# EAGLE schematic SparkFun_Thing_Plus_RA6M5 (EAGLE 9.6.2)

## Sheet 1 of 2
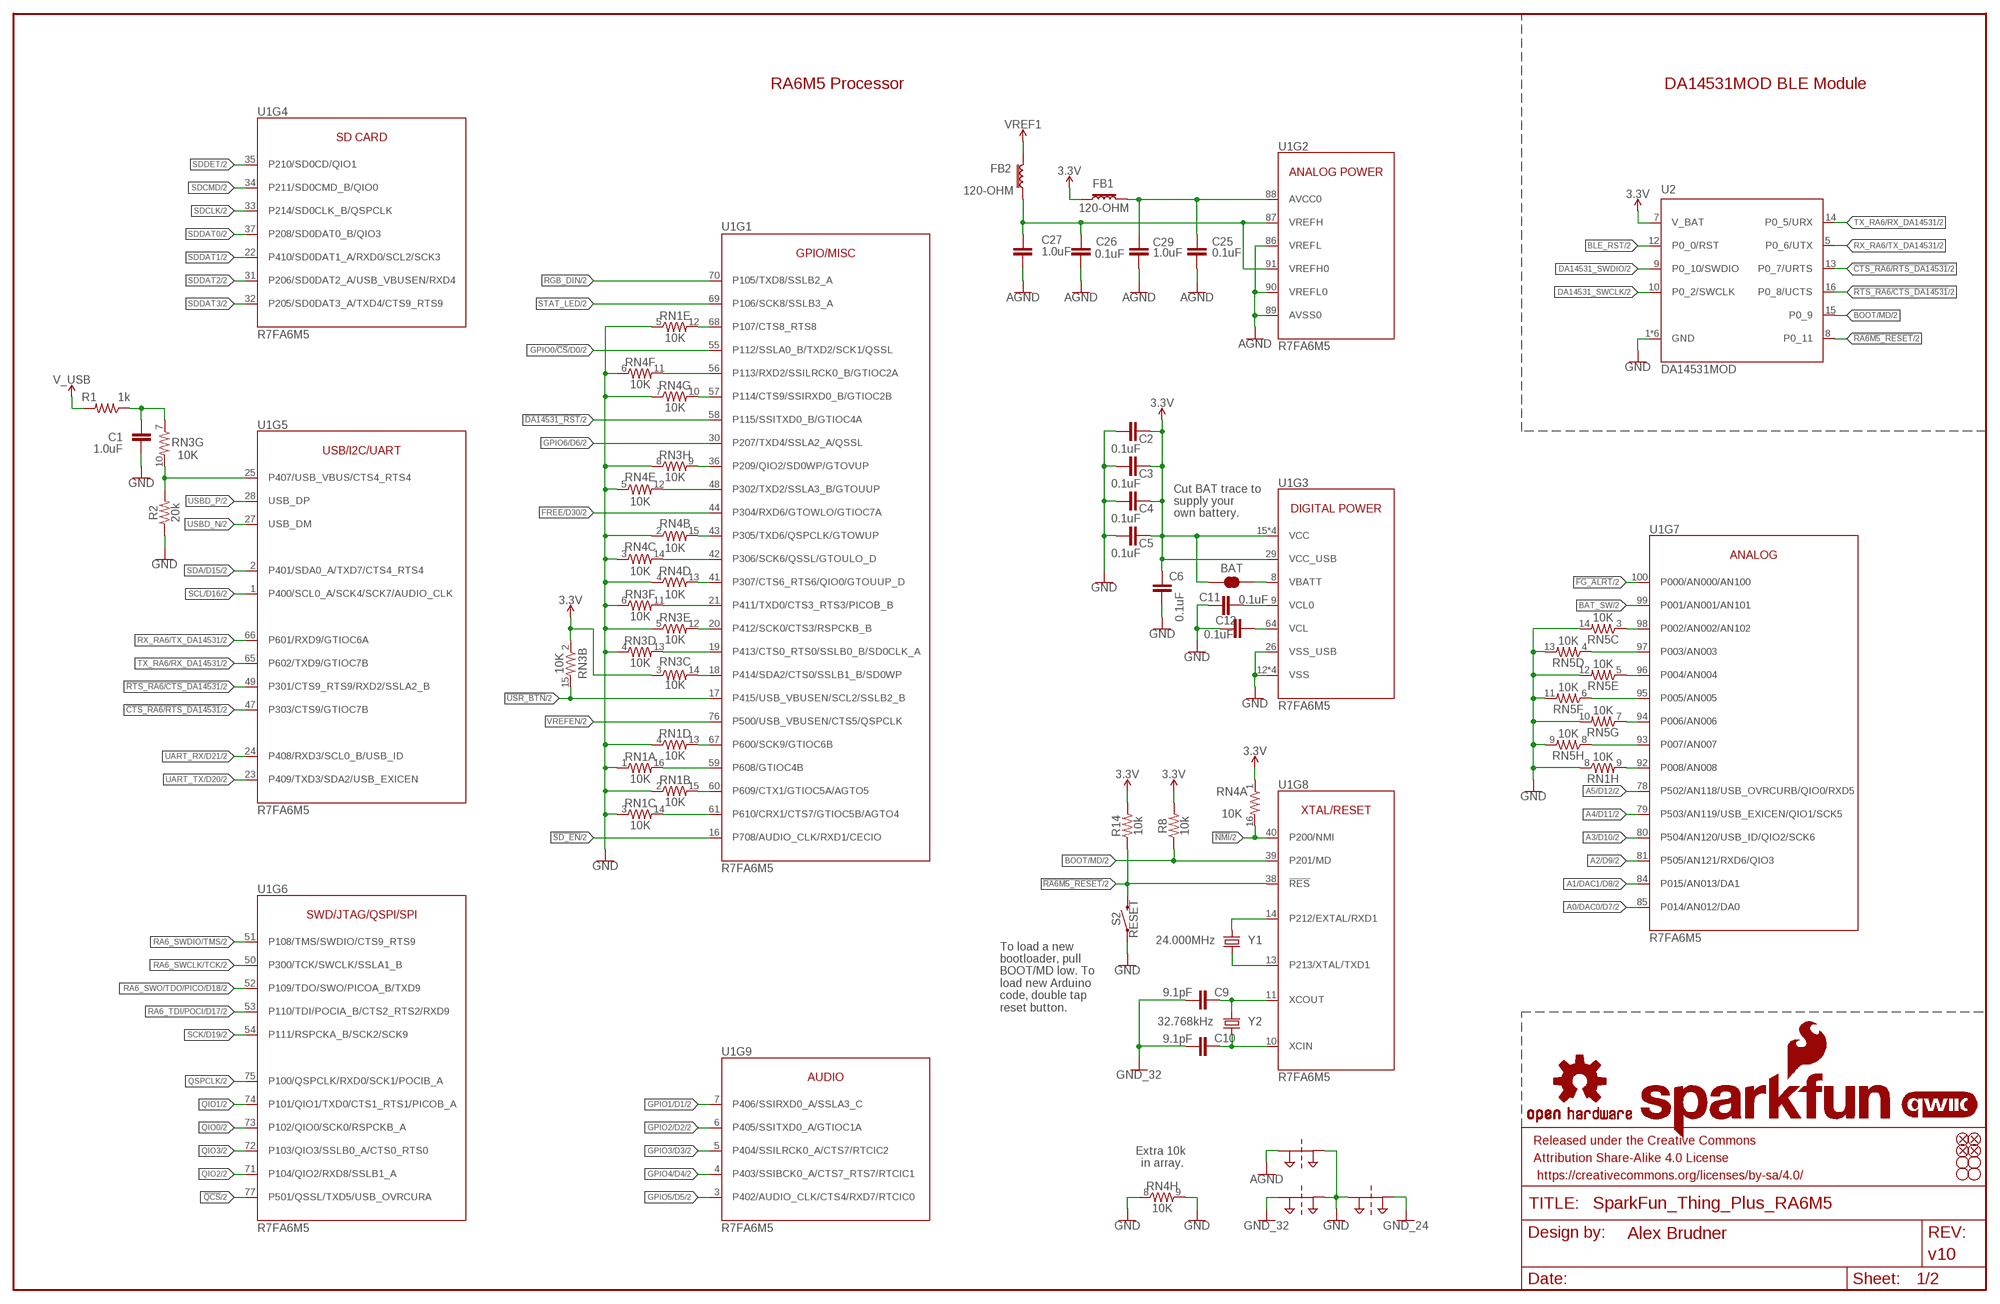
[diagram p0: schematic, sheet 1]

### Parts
BAT  JUMPER-SMT_2_NC_TRACE_SILK  [SMT-JUMPER_2_NC_TRACE_SILK]
C1  1.0uF  1.0UF-0402T-16V-10%  [0402-TIGHT]
C2  0.1uF  0.1UF-0402T-16V-10%  [0402-TIGHT]
C3  0.1uF  0.1UF-0402T-16V-10%  [0402-TIGHT]
C4  0.1uF  0.1UF-0402T-16V-10%  [0402-TIGHT]
C5  0.1uF  0.1UF-0402T-16V-10%  [0402-TIGHT]
C6  0.1uF  0.1UF-0402T-16V-10%  [0402-TIGHT]
C9  9.1pF  9.1PF-0402-TIGHT  [0402-TIGHT]
C10  9.1pF  9.1PF-0402-TIGHT  [0402-TIGHT]
C11  0.1uF  0.1UF-0402T-16V-10%  [0402-TIGHT]
C12  0.1uF  0.1UF-0402T-16V-10%  [0402-TIGHT]
C25  0.1uF  0.1UF-0402T-16V-10%  [0402-TIGHT]
C26  0.1uF  0.1UF-0402T-16V-10%  [0402-TIGHT]
C27  1.0uF  1.0UF-0402T-16V-10%  [0402-TIGHT]
C29  1.0uF  1.0UF-0402T-16V-10%  [0402-TIGHT]
FB1  120-OHM  FERRITE_BEAD-120_OHM-0402T  [0402-TIGHT]
FB2  120-OHM  FERRITE_BEAD-120_OHM-0402T  [0402-TIGHT]
FD1  FIDUCIALUFIDUCIAL  [FIDUCIAL-MICRO]
FD2  FIDUCIALUFIDUCIAL  [FIDUCIAL-MICRO]
FD3  FIDUCIALUFIDUCIAL  [FIDUCIAL-MICRO]
FD4  FIDUCIALUFIDUCIAL  [FIDUCIAL-MICRO]
FRAME1  FRAME-LEDGER  [CREATIVE_COMMONS]
H1  STAND-OFFTIGHT  [STAND-OFF-TIGHT]
H2  STAND-OFFTIGHT  [STAND-OFF-TIGHT]
H3  STAND-OFFTIGHT  [STAND-OFF-TIGHT]
H4  STAND-OFFTIGHT  [STAND-OFF-TIGHT]
LOGO1  OSHW-LOGOMINI  [OSHW-LOGO-MINI]
LOGO2  SFE_LOGO_NAME_FLAME.1_INCH  [SFE_LOGO_NAME_FLAME_.1]
LOGO3  QWIIC_LOGO_4MM  [QWIIC_4MM]
R1  1k  1KOHM-0402T-1/16W-1%  [0402-TIGHT]
R2  20k  20KOHM-0402T-1/16W-1%  [0402-TIGHT]
R8  10k  10KOHM-0402T-1/16W-1%  [0402-TIGHT]
R14  10k  10KOHM-0402T-1/16W-1%  [0402-TIGHT]
RN1  10K  10KOHM-ARRAY(8)-2506_ARV-1/16W-5%  [2506_AR]
RN3  10K  10KOHM-ARRAY(8)-2506_ARV-1/16W-5%  [2506_AR]
RN4  10K  10KOHM-ARRAY(8)-2506_ARV-1/16W-5%  [2506_AR]
RN5  10K  10KOHM-ARRAY(8)-2506_ARV-1/16W-5%  [2506_AR]
S2  RESET  MOMENTARY-SWITCH-SPST-SMD-4.6X2.8MM  [TACTILE_SWITCH_SMD_4.6X2.8MM]
SUPPLYTIE1  2PT_GND_TIESMALL  [2PT_GND_TIE_SMALL]
SUPPLYTIE2  2PT_GND_TIESMALL  [2PT_GND_TIE_SMALL]
SUPPLYTIE3  2PT_GND_TIESMALL  [2PT_GND_TIE_SMALL]
U1  R7FA6M5  R7FA6M5-100LQFP  [P-LQFP100-14X14-0.50]
U2  DA14531MOD  [DA14531MOD]
Y1  24.000MHz  CRYSTAL-24.000MHZ-8PF-4-SMD  [4-SMD,32X25]
Y2  32.768kHz  CRYSTAL-32.768KHZSMD-3.2X1.5  [CRYSTAL-SMD-3.2X1.5MM]

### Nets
3.3V [Power]: BAT.1 C2.1 C3.1 C4.1 C5.1 C6.1 FB1.1 R8.2 R14.2 RN3.2 RN3.3 RN4.1 U1.15(VCC) U1.29(VCC_USB) U1.46(VCC) U1.62(VCC) U1.82(VCC) U2.7(V_BAT) ; also sheet 2
!CTS_RA6/RTS_DA14531! [LS Digital]: U1.47(P303/CTS9/GTIOC7B) U2.13(P0_7/URTS) ; also sheet 2
!DA14531_RST!: U1.58(P115/SSITXD0_B/GTIOC4A) ; also sheet 2
!FG_ALRT!: U1.100(P000/AN000/AN100) ; also sheet 2
!NMI!: RN4.16 U1.40(P200/NMI) ; also sheet 2
!QCS!: U1.77(P501/QSSL/TXD5/USB_OVRCURA) ; also sheet 2
!RA6M5_RESET!: R14.1 S2.3 S2.4 U1.38(!RES!) U2.8(P0_11) ; also sheet 2
!RTS_RA6/CTS_DA14531! [LS Digital]: U1.49(P301/CTS9_RTS9/RXD2/SSLA2_B) U2.16(P0_8/UCTS) ; also sheet 2
!SD_EN!: U1.16(P708/AUDIO_CLK/RXD1/CECIO) ; also sheet 2
!USR_BTN!: RN3.15 U1.17(P415/USB_VBUSEN/SCL2/SSLB2_B) ; also sheet 2
A0/DAC0/D7 [Analog]: U1.85(P014/AN012/DA0) ; also sheet 2
A1/DAC1/D8 [Analog]: U1.84(P015/AN013/DA1) ; also sheet 2
A2/D9 [Analog]: U1.81(P505/AN121/RXD6/QIO3) ; also sheet 2
A3/D10 [Analog]: U1.80(P504/AN120/USB_ID/QIO2/SCK6) ; also sheet 2
A4/D11 [Analog]: U1.79(P503/AN119/USB_EXICEN/QIO1/SCK5) ; also sheet 2
A5/D12 [Analog]: U1.78(P502/AN118/USB_OVRCURB/QIO0/RXD5) ; also sheet 2
AGND [Analog Ground]: C25.2 C26.2 C27.2 C29.2 SUPPLYTIE1.P$1 U1.86(VREFL) U1.89(AVSS0) U1.90(VREFL0)
AVCC0 [Power]: C25.1 C29.1 FB1.2 U1.88(AVCC0) ; also sheet 2
BAT_SW: U1.99(P001/AN001/AN101) ; also sheet 2
BLE_RST: U2.12(P0_0/RST) ; also sheet 2
BOOT/MD: R8.1 U1.39(P201/MD) U2.15(P0_9) ; also sheet 2
DA14531_SWCLK [HS Digital]: U2.10(P0_2/SWCLK) ; also sheet 2
DA14531_SWDIO [HS Digital]: U2.9(P0_10/SWDIO) ; also sheet 2
EXTAL [CLK signals]: U1.14(P212/EXTAL/RXD1) Y1.1
FREE/D30: U1.44(P304/RXD6/GTOWLO/GTIOC7A) ; also sheet 2
GND [Power]: C1.1 C2.2 C3.2 C4.2 C5.2 C6.2 C11.2 C12.2 R2.1 RN1.1 RN1.2 RN1.3 RN1.4 RN1.5 RN1.8 RN3.4 RN3.5 RN3.6 RN3.8 RN4.2 RN4.3 RN4.4 RN4.5 RN4.6 RN4.7 RN4.8 RN4.9 RN5.9 RN5.10 RN5.11 RN5.12 RN5.13 RN5.14 S2.1 S2.2 SUPPLYTIE1.P$2 SUPPLYTIE2.P$2 SUPPLYTIE3.P$1 U1.12(VSS) U1.26(VSS_USB) U1.45(VSS) U1.63(VSS) U1.83(VSS) U2.1(GND) U2.2(GND) U2.3(GND) U2.4(GND) U2.6(GND) U2.11(GND) ; also sheet 2
GND_24 [CLK grounds]: SUPPLYTIE3.P$2
GND_32 [CLK grounds]: C9.1 C10.1 SUPPLYTIE2.P$1
GPIO0/!CS!/D0: U1.55(P112/SSLA0_B/TXD2/SCK1/QSSL) ; also sheet 2
GPIO1/D1: U1.7(P406/SSIRXD0_A/SSLA3_C) ; also sheet 2
GPIO2/D2: U1.6(P405/SSITXD0_A/GTIOC1A) ; also sheet 2
GPIO3/D3: U1.5(P404/SSILRCK0_A/CTS7/RTCIC2) ; also sheet 2
GPIO4/D4: U1.4(P403/SSIBCK0_A/CTS7_RTS7/RTCIC1) ; also sheet 2
GPIO5/D5: U1.3(P402/AUDIO_CLK/CTS4/RXD7/RTCIC0) ; also sheet 2
GPIO6/D6: U1.30(P207/TXD4/SSLA2_A/QSSL) ; also sheet 2
N$7: RN1.9 U1.92(P008/AN008)
N$8: RN3.9 U1.36(P209/QIO2/SD0WP/GTOVUP)
N$9: C1.2 R1.1 RN3.7
N$13: RN3.14 U1.18(P414/SDA2/CTS0/SSLB1_B/SD0WP)
N$15: R2.2 RN3.10 U1.25(P407/USB_VBUS/CTS4_RTS4)
N$17: RN1.14 U1.61(P610/CRX1/CTS7/GTIOC5B/AGTO4)
N$18: RN1.15 U1.60(P609/CTX1/GTIOC5A/AGTO5)
N$22: RN1.16 U1.59(P608/GTIOC4B)
N$23: RN4.15 U1.43(P305/TXD6/QSPCLK/GTOWUP)
N$24: RN1.13 U1.67(P600/SCK9/GTIOC6B)
N$26: RN3.13 U1.19(P413/CTS0_RTS0/SSLB0_B/SD0CLK_A)
N$27: RN3.12 U1.20(P412/SCK0/CTS3/RSPCKB_B)
N$28: RN3.11 U1.21(P411/TXD0/CTS3_RTS3/PICOB_B)
N$29 [Power]: C26.1 C27.1 FB2.1 U1.87(VREFH) U1.91(VREFH0)
N$30: RN4.13 U1.41(P307/CTS6_RTS6/QIO0/GTOUUP_D)
N$31: RN4.12 U1.48(P302/TXD2/SSLA3_B/GTOUUP)
N$32: RN4.14 U1.42(P306/SCK6/QSSL/GTOULO_D)
N$33 [Power]: BAT.2 U1.8(VBATT)
N$35: RN4.10 U1.57(P114/CTS9/SSIRXD0_B/GTIOC2B)
N$36: RN4.11 U1.56(P113/RXD2/SSILRCK0_B/GTIOC2A)
N$37: RN1.12 U1.68(P107/CTS8_RTS8)
N$41: RN5.8 U1.93(P007/AN007)
N$42: RN5.7 U1.94(P006/AN006)
N$43: RN5.6 U1.95(P005/AN005)
N$44: RN5.5 U1.96(P004/AN004)
N$45: RN5.4 U1.97(P003/AN003)
N$46: RN5.3 U1.98(P002/AN002/AN102)
N$97: C11.1 U1.9(VCL0)
N$98: C12.1 U1.64(VCL)
QIO0 [HS Digital]: U1.73(P102/QIO0/SCK0/RSPCKB_A) ; also sheet 2
QIO1 [HS Digital]: U1.74(P101/QIO1/TXD0/CTS1_RTS1/PICOB_A) ; also sheet 2
QIO2 [HS Digital]: U1.71(P104/QIO2/RXD8/SSLB1_A) ; also sheet 2
QIO3 [HS Digital]: U1.72(P103/QIO3/SSLB0_A/CTS0_RTS0) ; also sheet 2
QSPCLK [HS Digital]: U1.75(P100/QSPCLK/RXD0/SCK1/POCIB_A) ; also sheet 2
RA6_SWCLK/TCK [HS Digital]: U1.50(P300/TCK/SWCLK/SSLA1_B) ; also sheet 2
RA6_SWDIO/TMS [HS Digital]: U1.51(P108/TMS/SWDIO/CTS9_RTS9) ; also sheet 2
RA6_SWO/TDO/PICO/D18 [HS Digital]: U1.52(P109/TDO/SWO/PICOA_B/TXD9) ; also sheet 2
RA6_TDI/POCI/D17 [HS Digital]: U1.53(P110/TDI/POCIA_B/CTS2_RTS2/RXD9) ; also sheet 2
RGB_DIN [LS Digital]: U1.70(P105/TXD8/SSLB2_A) ; also sheet 2
RX_RA6/TX_DA14531 [LS Digital]: U1.66(P601/RXD9/GTIOC6A) U2.5(P0_6/UTX) ; also sheet 2
SCK/D19 [HS Digital]: U1.54(P111/RSPCKA_B/SCK2/SCK9) ; also sheet 2
SCL/D16 [LS Digital]: U1.1(P400/SCL0_A/SCK4/SCK7/AUDIO_CLK) ; also sheet 2
SDA/D15 [LS Digital]: U1.2(P401/SDA0_A/TXD7/CTS4_RTS4) ; also sheet 2
SDCLK [HS Digital]: U1.33(P214/SD0CLK_B/QSPCLK) ; also sheet 2
SDCMD [LS Digital]: U1.34(P211/SD0CMD_B/QIO0) ; also sheet 2
SDDAT0 [HS Digital]: U1.37(P208/SD0DAT0_B/QIO3) ; also sheet 2
SDDAT1 [HS Digital]: U1.22(P410/SD0DAT1_A/RXD0/SCL2/SCK3) ; also sheet 2
SDDAT2 [HS Digital]: U1.31(P206/SD0DAT2_A/USB_VBUSEN/RXD4) ; also sheet 2
SDDAT3 [HS Digital]: U1.32(P205/SD0DAT3_A/TXD4/CTS9_RTS9) ; also sheet 2
SDDET: U1.35(P210/SD0CD/QIO1) ; also sheet 2
STAT_LED: U1.69(P106/SCK8/SSLB3_A) ; also sheet 2
TX_RA6/RX_DA14531 [LS Digital]: U1.65(P602/TXD9/GTIOC7B) U2.14(P0_5/URX) ; also sheet 2
UART_RX/D21 [LS Digital]: U1.24(P408/RXD3/SCL0_B/USB_ID) ; also sheet 2
UART_TX/D20 [LS Digital]: U1.23(P409/TXD3/SDA2/USB_EXICEN) ; also sheet 2
USBD_N [USB diff]: U1.27(USB_DM) ; also sheet 2
USBD_P [USB diff]: U1.28(USB_DP) ; also sheet 2
V_USB [Power]: R1.2 ; also sheet 2
VREF1 [Power]: FB2.2 ; also sheet 2
VREFEN: U1.76(P500/USB_VBUSEN/CTS5/QSPCLK) ; also sheet 2
XCIN [CLK signals]: C10.2 U1.10(XCIN) Y2.P$1
XCOUT [CLK signals]: C9.2 U1.11(XCOUT) Y2.P$2
XTAL [CLK signals]: U1.13(P213/XTAL/TXD1) Y1.3

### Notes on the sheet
- RA6M5 Processor | DA14531MOD BLE Module
- Cut BAT trace to 
  supply your 
  own battery.
- To load a new 
  bootloader, pull 
  BOOT/MD low. To 
  load new Arduino 
  code, double tap 
  reset button.
- Extra 10k 
  in array.

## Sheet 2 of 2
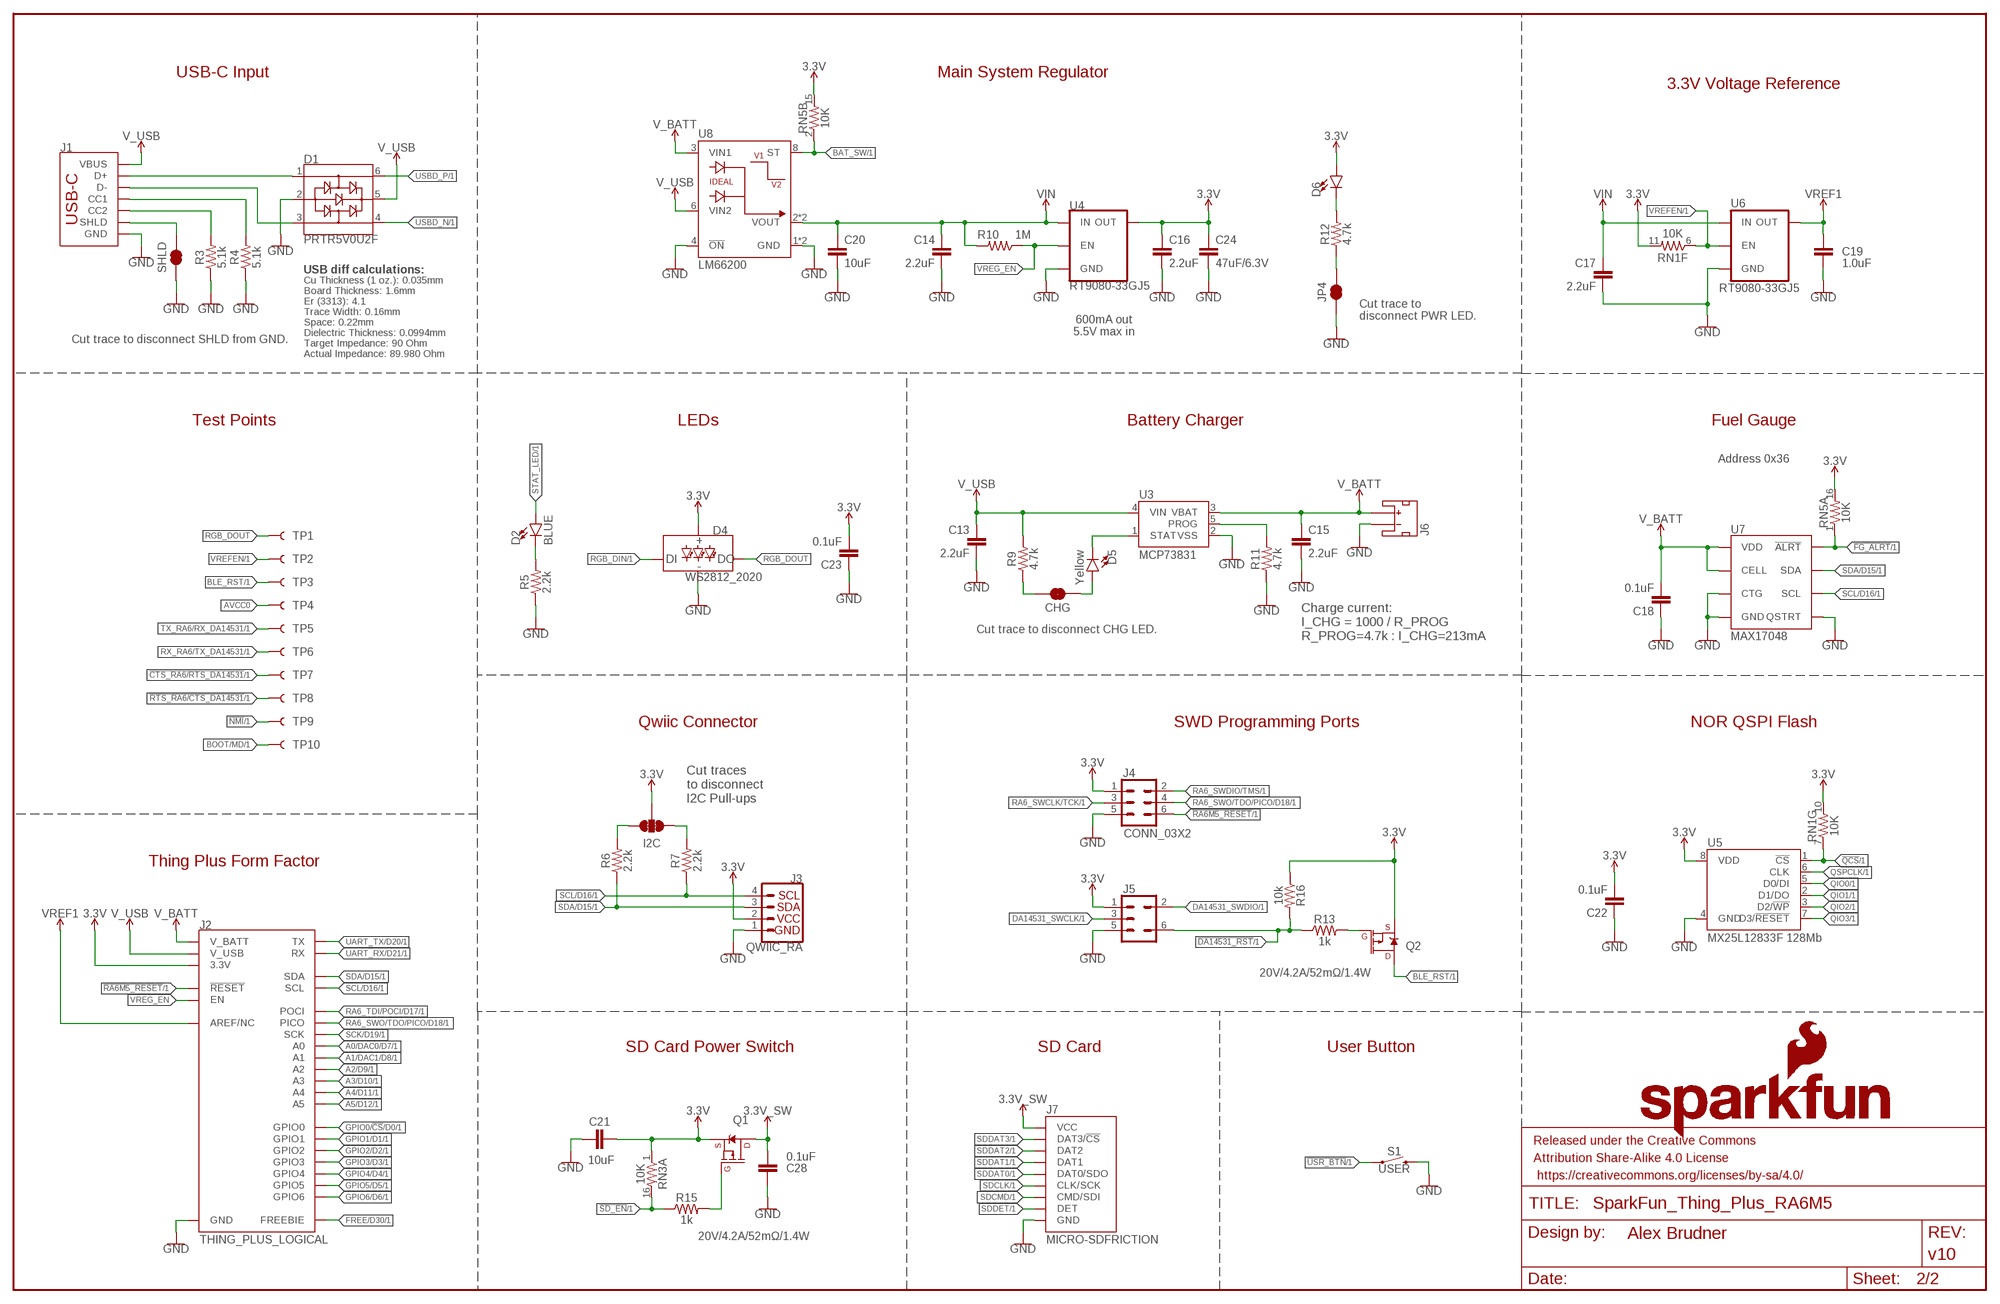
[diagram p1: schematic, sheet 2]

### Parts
C13  2.2uF  2.2UF-0402_TIGHT-10V-10%-X5R  [0402-TIGHT]
C14  2.2uF  2.2UF-0402_TIGHT-10V-10%-X5R  [0402-TIGHT]
C15  2.2uF  2.2UF-0402_TIGHT-10V-10%-X5R  [0402-TIGHT]
C16  2.2uF  2.2UF-0402_TIGHT-10V-10%-X5R  [0402-TIGHT]
C17  2.2uF  2.2UF-0402_TIGHT-10V-10%-X5R  [0402-TIGHT]
C18  0.1uF  0.1UF-0402T-16V-10%  [0402-TIGHT]
C19  1.0uF  1.0UF-0402T-16V-10%  [0402-TIGHT]
C20  10uF  10UF-0805-25V-10%  [0805]
C21  10uF  10UF-0805-25V-10%  [0805]
C22  0.1uF  0.1UF-0402T-16V-10%  [0402-TIGHT]
C23  0.1uF  0.1UF-0402T-16V-10%  [0402-TIGHT]
C24  47uF/6.3V  47UF  [0805]
C28  0.1uF  0.1UF-0402T-16V-10%  [0402-TIGHT]
CHG  JUMPER-SMT_2_NC_TRACE_SILK  [SMT-JUMPER_2_NC_TRACE_SILK]
D1  PRTR5V0U2F  [SOT886]
D2  BLUE  LED-BLUE0603  [LED-0603]
D4  WS2812_2020  [WS2812-2020]
D5  Yellow  LED-YELLOW0603  [LED-0603]
D6  LED-RED_0603-KB  [LED-0603]
FRAME2  FRAME-LEDGERNO_FOOTPRINT  [DUMMY]
I2C  JUMPER-SMT_3_2-NC_TRACE_SILK  [SMT-JUMPER_3_2-NC_TRACE_SILK]
J1  USB Female Type C Connector  USB_C_6-LAYER-ISOLATED  [USB-C-16P-6LAYER-ISOLATED]
J2  THING_PLUS_LOGICAL  [THING_PLUS]
J3  QWIIC_RA  QWIIC_CONNECTORJS-1MM  [JST04_1MM_RA]
J4  CONN_03X2  [PAD_05_03X2_TP]
J5  SWD-5PIN  [PAD_05_03X2_TP_NO4]
J6  JST_2MM_MALE  [JST-2-SMD]
J7  MICRO-SDFRICTION  [MICROSD_TINY]
JP4  JUMPER-SMT_2_NC_TRACE_SILK  [SMT-JUMPER_2_NC_TRACE_SILK]
LOGO4  SFE_LOGO_NAME_FLAMEBLANK  [BLANK]
Q1  20V/4.2A/52mΩ/1.4W  MOSFET_PCH-DMG2305UX-7  [SOT23-3]
Q2  20V/4.2A/52mΩ/1.4W  MOSFET_PCH-DMG2305UX-7  [SOT23-3]
R3  5.1k  5.1KOHM-0402T-1/16W-1%  [0402-TIGHT]
R4  5.1k  5.1KOHM-0402T-1/16W-1%  [0402-TIGHT]
R5  2.2k  2.2KOHM-0402T-1/16W-1%  [0402-TIGHT]
R6  2.2k  2.2KOHM-0402T-1/16W-1%  [0402-TIGHT]
R7  2.2k  2.2KOHM-0402T-1/16W-1%  [0402-TIGHT]
R9  4.7k  4.7KOHM-0402T-1/16W-1%  [0402-TIGHT]
R10  1M  1MOHM-0402T-1/16W-5%  [0402-TIGHT]
R11  4.7k  4.7KOHM-0402T-1/16W-1%  [0402-TIGHT]
R12  4.7k  4.7KOHM-0402T-1/16W-1%  [0402-TIGHT]
R13  1k  1KOHM-0402T-1/16W-1%  [0402-TIGHT]
R15  1k  1KOHM-0402T-1/16W-1%  [0402-TIGHT]
R16  10k  10KOHM-0402T-1/16W-1%  [0402-TIGHT]
S1  USER  MOMENTARY-SWITCH-SPST-SMD-4.6X2.8MM  [TACTILE_SWITCH_SMD_4.6X2.8MM]
SHLD  JUMPER-SMT_2_NC_TRACE_SILK  [SMT-JUMPER_2_NC_TRACE_SILK]
TP1  TEST-POINT3X5  [PAD.03X.05]
TP2  TEST-POINT3X4  [PAD.03X.04]
TP3  TEST-POINT3X5  [PAD.03X.05]
TP4  TEST-POINT3  [PAD.03X.03]
TP5  TEST-POINT3X5  [PAD.03X.05]
TP6  TEST-POINT3X5  [PAD.03X.05]
TP7  TEST-POINT3X5  [PAD.03X.05]
TP8  TEST-POINT3X5  [PAD.03X.05]
TP9  TEST-POINT3  [PAD.03X.03]
TP10  TEST-POINT3X5  [PAD.03X.05]
U3  MCP73831  [SOT23-5]
U4  RT9080-33GJ5  V_REG_RT9080  [SOT23-5]
U5  MX25L12833F 128Mb  MX25L12833F_128MBIT_QSPI  [WSON-8-6X5]
U6  RT9080-33GJ5  V_REG_RT9080  [SOT23-5]
U7  MAX17048  MAX17048DFN8  [DFN-8]
U8  LM66200  IDEAL_DIODE_DUAL_LM66200  [SOT8]

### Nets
3.3V [Power]: C16.1 C21.1 C22.2 C23.2 C24.1 D4.VCC D6.A I2C.2 J2.27(3.3V) J3.2 J4.1 J5.1 Q1.2(S) Q2.2(S) R16.1 RN1.10 RN1.11 RN3.1 RN5.15 RN5.16 U4.5(OUT) U5.8(VDD) ; also sheet 1
3.3V_SW [Power]: C28.2 J7.4(VCC) Q1.3(D)
!CTS_RA6/RTS_DA14531! [LS Digital]: TP7.1 ; also sheet 1
!DA14531_RST!: J5.6 R13.1 R16.2 ; also sheet 1
!FG_ALRT!: RN5.1 U7.5(!ALRT) ; also sheet 1
!NMI!: TP9.1 ; also sheet 1
!QCS!: RN1.7 U5.1(!CS!) ; also sheet 1
!RA6M5_RESET!: J2.28(!RESET) J4.6 ; also sheet 1
!RTS_RA6/CTS_DA14531! [LS Digital]: TP8.1 ; also sheet 1
!SD_EN!: R15.1 RN3.16 ; also sheet 1
!USR_BTN!: S1.1 S1.2 ; also sheet 1
A0/DAC0/D7 [Analog]: J2.24(A0) ; also sheet 1
A1/DAC1/D8 [Analog]: J2.23(A1) ; also sheet 1
A2/D9 [Analog]: J2.22(A2) ; also sheet 1
A3/D10 [Analog]: J2.21(A3) ; also sheet 1
A4/D11 [Analog]: J2.20(A4) ; also sheet 1
A5/D12 [Analog]: J2.19(A5) ; also sheet 1
AVCC0 [Power]: TP4.1 ; also sheet 1
BAT_SW: RN5.2 U8.8(ST) ; also sheet 1
BLE_RST: Q2.3(D) TP3.1 ; also sheet 1
BOOT/MD: TP10.1 ; also sheet 1
DA14531_SWCLK [HS Digital]: J5.3 ; also sheet 1
DA14531_SWDIO [HS Digital]: J5.2 ; also sheet 1
FREE/D30: J2.13(FREEBIE) ; also sheet 1
GND [Power]: C13.2 C14.2 C15.2 C16.2 C17.2 C18.1 C19.2 C20.2 C21.2 C22.1 C23.1 C24.2 C28.1 D1.2 D4.GND J1.GND J1.GND2(GND) J2.25(GND) J3.1 J4.5 J5.5 J6.1(-) J7.6(GND) J7.GND1(GND) J7.GND2(GND) J7.GND3(GND) J7.GND4(GND) J7.GND5(GND) J7.GND6(GND) JP4.1 R3.1 R4.1 R5.1 R11.1 S1.3 S1.4 SHLD.1 U3.2(VSS) U4.2(GND) U5.4(GND) U6.2(GND) U7.1(CTG) U7.4(GND) U7.6(QSTRT) U7.9(GND) U8.1(GND) U8.4(!ON!) U8.5(GND) ; also sheet 1
GPIO0/!CS!/D0: J2.9(GPIO0) ; also sheet 1
GPIO1/D1: J2.8(GPIO1) ; also sheet 1
GPIO2/D2: J2.7(GPIO2) ; also sheet 1
GPIO3/D3: J2.6(GPIO3) ; also sheet 1
GPIO4/D4: J2.5(GPIO4) ; also sheet 1
GPIO5/D5: J2.4(GPIO5) ; also sheet 1
GPIO6/D6: J2.3(GPIO6) ; also sheet 1
N$1: CHG.2 R9.1
N$2: CHG.1 D5.A
N$3: D5.C U3.1(STAT)
N$4: Q2.1(G) R13.2
N$5: R11.2 U3.5(PROG)
N$6: D2.C R5.2
N$10: I2C.1 R6.2
N$11: I2C.3 R7.2
N$14: JP4.2 R12.1
N$16: D6.C R12.2
N$19: J1.SHLD1(SHLD) J1.SHLD2(SHLD) J1.SHLD3(SHLD) J1.SHLD4(SHLD) J1.SHLD5(SHLD) J1.SHLD6(SHLD) J1.SHLD7(SHLD) J1.SHLD8(SHLD) SHLD.2
N$20: J1.B5(CC2) R3.2
N$21: J1.A5(CC1) R4.2
N$47: Q1.1(G) R15.2
QIO0 [HS Digital]: U5.5(D0/DI) ; also sheet 1
QIO1 [HS Digital]: U5.2(D1/DO) ; also sheet 1
QIO2 [HS Digital]: U5.3(D2/!WP!) ; also sheet 1
QIO3 [HS Digital]: U5.7(D3/!RESET!) ; also sheet 1
QSPCLK [HS Digital]: U5.6(CLK) ; also sheet 1
RA6_SWCLK/TCK [HS Digital]: J4.3 ; also sheet 1
RA6_SWDIO/TMS [HS Digital]: J4.2 ; also sheet 1
RA6_SWO/TDO/PICO/D18 [HS Digital]: J2.17(PICO) J4.4 ; also sheet 1
RA6_TDI/POCI/D17 [HS Digital]: J2.16(POCI) ; also sheet 1
RGB_DIN [LS Digital]: D4.DI ; also sheet 1
RGB_DOUT [LS Digital]: D4.DO TP1.1
RX_RA6/TX_DA14531 [LS Digital]: TP6.1 ; also sheet 1
SCK/D19 [HS Digital]: J2.18(SCK) ; also sheet 1
SCL/D16 [LS Digital]: J2.2(SCL) J3.4 R7.1 U7.7(SCL) ; also sheet 1
SDA/D15 [LS Digital]: J2.1(SDA) J3.3 R6.1 U7.8(SDA) ; also sheet 1
SDCLK [HS Digital]: J7.5(CLK/SCK) ; also sheet 1
SDCMD [LS Digital]: J7.3(CMD/SDI) ; also sheet 1
SDDAT0 [HS Digital]: J7.7(DAT0/SDO) ; also sheet 1
SDDAT1 [HS Digital]: J7.8(DAT1) ; also sheet 1
SDDAT2 [HS Digital]: J7.1(DAT2) ; also sheet 1
SDDAT3 [HS Digital]: J7.2(DAT3/!CS!) ; also sheet 1
SDDET: J7.9(DET) ; also sheet 1
STAT_LED: D2.A ; also sheet 1
TX_RA6/RX_DA14531 [LS Digital]: TP5.1 ; also sheet 1
UART_RX/D21 [LS Digital]: J2.15(RX) ; also sheet 1
UART_TX/D20 [LS Digital]: J2.14(TX) ; also sheet 1
USBD_N [USB diff]: D1.4 ; also sheet 1
USBD_P [USB diff]: D1.6 ; also sheet 1
USBIN_N [USB diff]: D1.3 J1.A7(D-) J1.B7(D-)
USBIN_P [USB diff]: D1.1 J1.A6(D+) J1.B6(D+)
V_BATT [Power]: C15.1 C18.2 J2.12(V_BATT) J6.2(+) U3.3(VBAT) U7.2(CELL) U7.3(VDD) U8.3(VIN1)
V_USB [Power]: C13.1 D1.5 J1.VBUS1(VBUS) J1.VBUS2(VBUS) J2.10(V_USB) R9.2 U3.4(VIN) U8.6(VIN2) ; also sheet 1
VIN [Power]: C14.1 C17.1 C20.1 R10.2 U4.1(IN) U6.1(IN) U8.2(VOUT) U8.7(VOUT)
VREF1 [Power]: C19.1 J2.26(AREF/NC) U6.5(OUT) ; also sheet 1
VREFEN: RN1.6 TP2.1 U6.3(EN) ; also sheet 1
VREG_EN: J2.11(EN) R10.1 U4.3(EN)
Unconnected: J6.NC1(PAD1) J6.NC2(PAD2)

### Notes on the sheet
- USB-C Input | Main System Regulator
- 3.3V Voltage Reference
- USB diff calculations:
- Cu Thickness (1 oz.): 0.035mm
  Board Thickness: 1.6mm
  Er (3313): 4.1
  Trace Width: 0.16mm
  Space: 0.22mm
  Dielectric Thickness: 0.0994mm
  Target Impedance: 90 Ohm
  Actual Impedance: 89.980 Ohm
- 600mA out
  5.5V max in
- Cut trace to 
  disconnect PWR LED.
- Cut trace to disconnect SHLD from GND.
- Test Points | LEDs | Battery Charger | Fuel Gauge
- Address 0x36
- Cut trace to disconnect CHG LED.
- Charge current:
  I_CHG = 1000 / R_PROG
  R_PROG=4.7k : I_CHG=213mA
- Qwiic Connector | SWD Programming Ports | NOR QSPI Flash
- Cut traces 
  to disconnect 
  I2C Pull-ups
- Thing Plus Form Factor
- SD Card Power Switch | SD Card | User Button

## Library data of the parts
BAT CHG JP4 SHLD = SparkFun-Jumpers:JUMPER-SMT_2_NC_TRACE: Normally closed trace jumper
C1 C19 C27 C29 = SparkFun-Capacitors:1.0UF: 1µF ceramic capacitors; PROD_ID: CAP-12417
C2-C6 C11 C12 C18 C22 C23 C25 C26 C28 = SparkFun-Capacitors:0.1UF: 0.1µF ceramic capacitors; PROD_ID: CAP-12416
C9 C10 = SparkFun-Capacitors:9.1PF: 9.1pF ceramic capacitors; MOUSER_PART: 609-500R07S9R1CV4T; PROD_ID: CAP-15278
C13-C17 = SparkFun-Capacitors:2.2UF: 2.2µF ceramic capacitors; PROD_ID: CAP-14232
C20 C21 = SparkFun-Capacitors:10UF: 10.0µF ceramic capacitors; PROD_ID: CAP-14259
C24 = SparkFun-Capacitors:47UF; PROD_ID: CAP-13854
D1 = SparkFun-IC-Power:PRTR5V0U2: A small ESD protection device. Most commonly used on USB D+/D- signals to protect large, expensive, or especially sensitive USB enabled devices.; PROD_ID: DIO-14084
D2 = SparkFun-LED:LED-BLUE: Blue SMD LED; PROD_ID: DIO-08575
D4 = SparkFun-LED:WS2812: Addressable RGB LED - 1 Wire Common names: WS2812, SK6812, Neopixel, APA-106, etc. SMD LED with built-in controller IC. Color: Red/Green/Blue SparkFun Products: LED-SMD RGB (WS2812) LED - RGB Addressable, PTH, 5mm Diffused (5 Pack) LED - RGB Addressable, PTH, 5mm Clear (5 Pack) Blynk Board -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; PROD_ID: DIO-15591
D5 = SparkFun-LED:LED-YELLOW: Yellow SMD LED; PROD_ID: DIO-09003
D6 = SparkFun-LED:LED-RED: Red SMD LED; PROD_ID: DIO-17976
FB1 FB2 = SparkFun-Coils:FERRITE_BEAD-120_OHM: Ferrite Bead (blocks, cores, rings, chokes, etc.); PROD_ID: NDUC-14206
FD1-FD4 = SparkFun-Aesthetics:FIDUCIAL: Fiducial Alignment Points
FRAME1 FRAME2 = SparkFun-Aesthetics:FRAME-LEDGER: Schematic Frame - Ledger; DESIGNER: Alex Brudner; REV: v10
H1-H4 = SparkFun-Hardware:STAND-OFF: Stand Off
I2C = SparkFun-Jumpers:JUMPER-SMT_3_2-NC_TRACE: Normally closed trace jumper (2 of 2 connections) This jumper has a trace between all three pads so they are normally closed (NC). Use a razor knife to open the connection(s). For best results follow the IPC guidelines for cutting traces: Cutout at least 0.063 mm (0.005 in). Remove all loose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
J1 = SparkFun_Thing_Plus_RA6M5:USB_C: USB Type C 16Pin Connector Super Speed pins not available on the 16-pin purely SMD connector so this part is best for USB 2.0 implementations. D1 and D2 are tied together enabling D+/- no matter which way the cable is plugged into the connector. The two channel configuration pins (CC1/2) are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; PROD_ID: CONN-14122
J2 = SparkFun-Boards:THING_PLUS_LOGICAL
J3 = SparkFun-Connectors:QWIIC_CONNECTOR: SparkFun I2C Standard Qwiic Connector An SMD 1mm pitch JST connector makes it easy and quick (get it? Qwiic?) to connect I2C devices to each other. The Qwiic system enables fast and solderless connection between popular platforms and various sensors and actuators. We carry 200mm, 100mm, 50mm, and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; PROD_ID: CONN-13694; VALUE: QWIIC_RIGHT_ANGLE
J4 = SparkFun_Thing_Plus_RA6M5:CONN_03X2
J5 = SparkFun-Connectors:SWD-5PIN: 5-pin SWD connector Test-point based header for SWD. Pin 1 - PWR Pin 2 - SWDIO Pin 3 - SWCLK Pin 4 - NC Pin 5 - GND Pin 6 - RESET
J6 = SparkFun-Connectors:JST_2MM_MALE: JST 2MM MALE RA CONNECTOR Two pin, compact surface mount connector. Commonly used as a battery input connection point. We really like the solid locking feeling and high current rating on these small connectors. We use these all the time as battery connectors. Mates to single-cell LiPo batteries.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; PROD_ID: CONN-11443; SF_ID: PRT-08612
J7 = SparkFun-Connectors:MICRO-SD: microSD Socket for Transflash Various sockets for µSD. tDoc lines correctly indicate media card edge positions when inserting (unlocked, locked, depressed). NOTE: CD1 and CD2 are connected internally, and the default detect state of the socket is detect pin to ground. SparkFun Products: WAV Trigger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; PROD_ID: CONN-13500
LOGO1 = SparkFun-Aesthetics:OSHW-LOGO: Open-Source Hardware (OSHW) Logo
LOGO2 LOGO4 = SparkFun-Aesthetics:SFE_LOGO_NAME_FLAME: SparkFun Font Logo w/ Flame
LOGO3 = SparkFun-Aesthetics:QWIIC_LOGO: Qwiic Logos for placement on schematic and PCB. The 5.5mm silk logo is best for placing next to Qwiic connector.
Q1 Q2 = SparkFun-DiscreteSemi:MOSFET_PCH: P-channel MOSFETs Voltage controlled devices that allow control of high current outputs. SparkFun Products: SparkFun ESP32 Thing SparkFun ESP8266 Thing SparkFun Pi Servo HAT V2 DMG2305UX-7 (20V/4.2A/SOT23-3); PROD_ID: TRANS-14388
R1 R13 R15 = SparkFun-Resistors:1KOHM: 1kΩ resistor; PROD_ID: RES-14342
R2 = SparkFun-Resistors:20KOHM: 20kΩ resistor; PROD_ID: RES-15131
R3 R4 = SparkFun-Resistors:5.1KOHM; PROD_ID: RES-14340
R5-R7 = SparkFun-Resistors:2.2KOHM: 2.2kΩ resistor; PROD_ID: RES-14341
R8 R14 R16 = SparkFun-Resistors:10KOHM: 10kΩ resistor; PROD_ID: RES-14241
R9 R11 R12 = SparkFun-Resistors:4.7KOHM: 4.7kΩ resistor; PROD_ID: RES-15343
R10 = SparkFun-Resistors:1MOHM: 1MΩ resistor; PROD_ID: RES-15185
RN1 RN3-RN5 = SparkFun_Thing_Plus_RA6M5:10KOHM-ARRAY(8)-2506_ARV-1/16W-5%; PROD_ID: RES-14952
S1 S2 = SparkFun-Switches:MOMENTARY-SWITCH-SPST: Momentary Switch (Pushbutton) - SPST; PROD_ID: SWCH-15606
SUPPLYTIE1-SUPPLYTIE3 = SparkFun_Thing_Plus_RA6M5:2PT_GND_TIE: Dual Ground Supply
TP1-TP10 = SparkFun-Connectors:TEST-POINT: SparkFun Test Points
U1 = SparkFun_Thing_Plus_RA6M5:R7FA6M5-100LQFP; PROD_ID: IC-20781
U2 = SparkFun_Thing_Plus_RA6M5:DA14531MOD; PROD_ID: IC-20782
U3 = SparkFun-IC-Power:MCP73831: MCP73831T Li-Ion, Li-Pol Controller Miniature single cell, fully integrated Li-Ion, Li-polymer charge management controller Datasheet SparkFun Products: SparkFun ESP32 Thing SparkFun 9DoF Razor IMU M0; PROD_ID: IC-09995
U4 U6 = SparkFun-IC-Power:V_REG_RT9080; PROD_ID: VREG-19034
U5 = SparkFun-IC-Memory:MX25L12833F_128MBIT_QSPI: Macronix MX25L12833FZNI-10G 128MBit QSPI MX25L12833F is 128Mb bits Serial NOR Flash memory.; PN: MX25L12833F-10G; PROD_ID: IC-21738
U7 = SparkFun-IC-Power:MAX17048: Micropower 1-Cell Li+ ModelGauge SparkFun Products Qduino Mini (DEV-13614); PROD_ID: IC-12551
U8 = SparkFun_Thing_Plus_RA6M5:IDEAL_DIODE_DUAL_LM66200; PROD_ID: IC-20783
Y1 = SparkFun_Thing_Plus_RA6M5:CRYSTAL-24.000MHZ-8PF-4-SMD; PN: RH100-24.000-8-1015-EXT-TR-NS1; PROD_ID: XTAL-20784
Y2 = SparkFun-Clocks:CRYSTAL-32.768KHZ: 32.768kHz Crystal; PROD_ID: XTAL-13062

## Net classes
2 CLK signals: width 0.15 mm, drill 0.2 mm, clearance 0.15 mm to class 0, clearance 0.15 mm to class 1, clearance 0.15 mm
3 Analog Ground: width 0.2 mm, clearance 0.2 mm to class 1, clearance 0.3 mm to class 2
4 Power: width 0.2 mm, drill 0.3 mm, clearance 0.2 mm to class 0, clearance 0.1 mm to class 1, clearance 0.15 mm to class 2, clearance 0.2 mm to class 3, clearance 0.2 mm
5 USB diff: width 0.16 mm, drill 0.2 mm, clearance 0.3 mm to class 0, clearance 0.3 mm to class 1, clearance 0.3 mm to class 2, clearance 0.3 mm to class 3, clearance 0.2 mm to class 4, clearance 0.22 mm

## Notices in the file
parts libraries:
SparkFun-Aesthetics: Licensing: Creative Commons ShareAlike 4.0 International - https://creativecommons.org/licenses/by-sa/4.0
SparkFun-Aesthetics: Released under the Creative Commons Attribution Share-Alike 4.0 License
SparkFun-Aesthetics: https://creativecommons.org/licenses/by-sa/4.0
